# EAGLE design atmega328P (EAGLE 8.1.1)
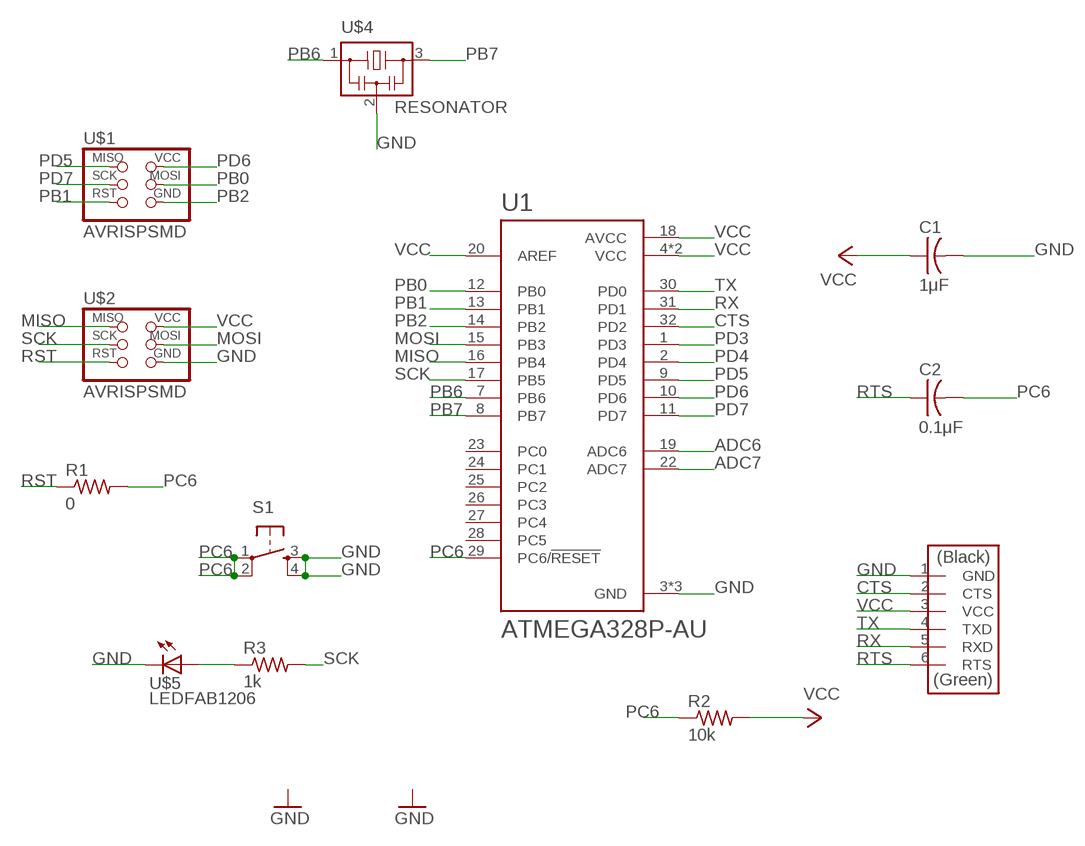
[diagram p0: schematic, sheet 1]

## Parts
C1  1μF  CAP-US1206FAB  [C1206FAB]
C2  0.1μF  CAP-US1206FAB  [C1206FAB]
R1  0  RES-US1206FAB  [R1206FAB]
R2  10k  RES-US1206FAB  [R1206FAB]
R3  1k  RES-US1206FAB  [R1206FAB]
S1  6MM_SWITCH6MM_SWITCH  [6MM_SWITCH]
U1  ATMEGA328P-AU  [QFP80P900X900X120-32N]
U$1  AVRISPSMD  [2X03SMD]
U$2  AVRISPSMD  [2X03SMD]
U$3  FTDI-SMD-HEADER  [1X06SMD]
U$4  RESONATOR  [EFOBM]
U$5  LEDFAB1206  [LED1206FAB]

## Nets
ADC6: U1.19(ADC6)
ADC7: U1.22(ADC7)
CTS: U1.32(PD2) U$3.2(CTS)
GND: C1.2 S1.3(S) S1.4(S1) U1.3(GND) U1.5(GND) U1.21(GND) U$2.6(GND) U$3.1(GND) U$4.2 U$5.2(C)
MISO: U1.16(PB4) U$2.1(MISO)
MOSI: U1.15(PB3) U$2.4(MOSI)
N$1: R3.1 U$5.1(A)
PB0: U1.12(PB0) U$1.4(MOSI)
PB1: U1.13(PB1) U$1.5(RST)
PB2: U1.14(PB2) U$1.6(GND)
PB6: U1.7(PB6) U$4.1
PB7: U1.8(PB7) U$4.3
PC6: C2.2 R1.2 R2.1 S1.1(P) S1.2(P1) U1.29(PC6/!RESET)
PD3: U1.1(PD3)
PD4: U1.2(PD4)
PD5: U1.9(PD5) U$1.1(MISO)
PD6: U1.10(PD6) U$1.2(VCC)
PD7: U1.11(PD7) U$1.3(SCK)
RST: R1.1 U$2.5(RST)
RTS: C2.1 U$3.6(RTS)
RX: U1.31(PD1) U$3.5(RXD)
SCK: R3.2 U1.17(PB5) U$2.3(SCK)
TX: U1.30(PD0) U$3.4(TXD)
VCC: C1.1 R2.2 U1.4(VCC) U1.6(VCC) U1.18(AVCC) U1.20(AREF) U$2.2(VCC) U$3.3(VCC)
Unconnected: U1.23(PC0) U1.24(PC1) U1.25(PC2) U1.26(PC3) U1.27(PC4) U1.28(PC5)

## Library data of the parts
C1 C2 = fab:CAP-US
R1-R3 = fab:RES-US: Resistor (US Symbol)
S1 = fab:6MM_SWITCH: OMRON SWITCH
U1 = ATMEGA328P-AU:ATMEGA328P-AU: ATmega Series 20 MHz 32 KB Flash 2 KB SRAM 8-Bit Microcontroller - TQFP-32; AVAILABILITY: Good; DESCRIPTION: ATmega Series 20 MHz 32 KB Flash 2 KB SRAM 8-Bit Microcontroller - TQFP-32; MF: Atmel; MP: ATMEGA328P-AU; PACKAGE: TQFP-32 Atmel; PRICE: 2.40 USD
U$1 U$2 = fab:AVRISP
U$3 = fab:FTDI-SMD-HEADER
U$4 = fab:RESONATOR
U$5 = fab:LED: LED

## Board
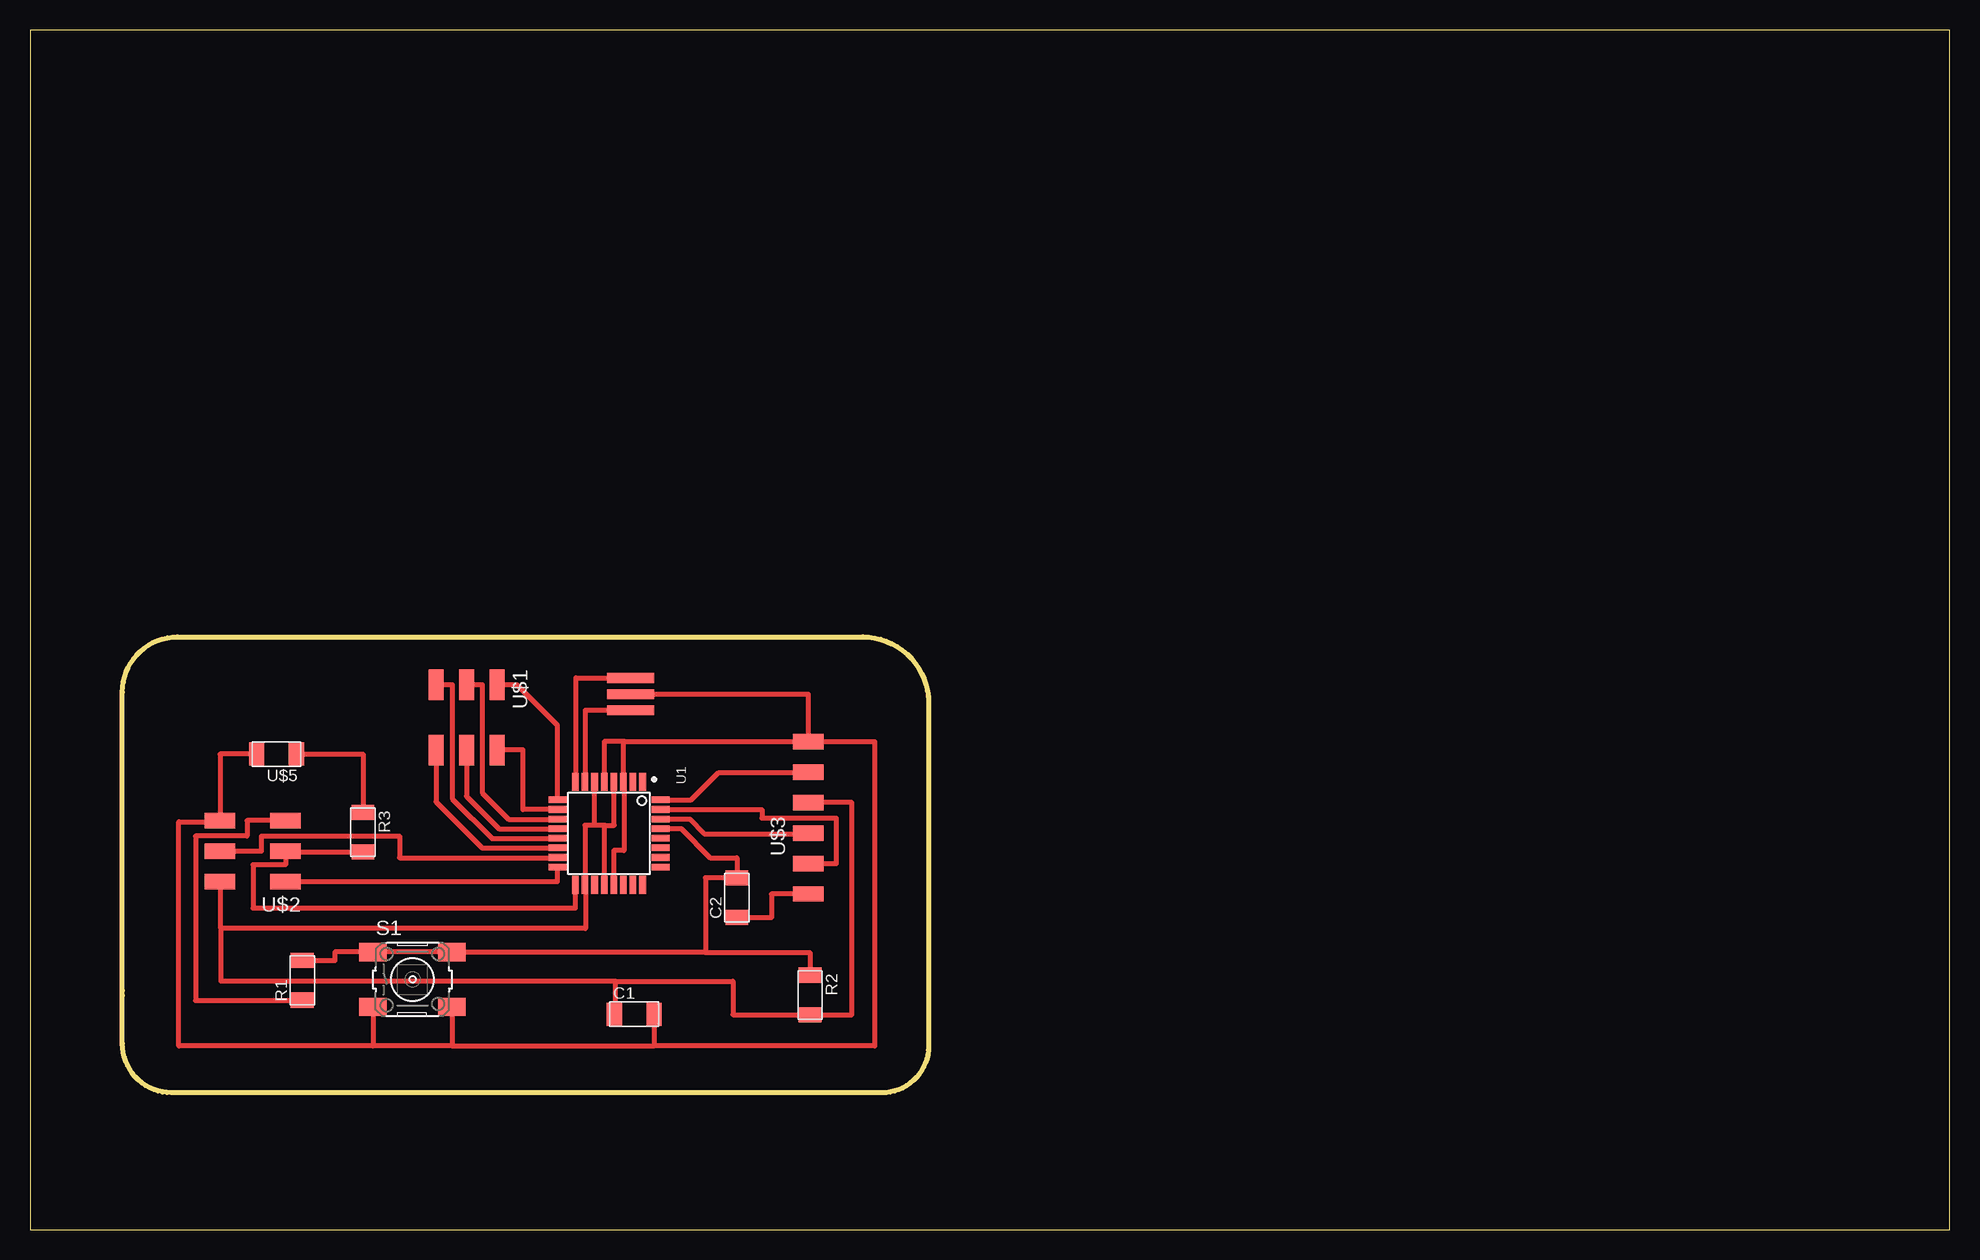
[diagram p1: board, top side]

Size 160 x 100 mm. Coordinates in mm from the lower left corner, seen from the top.
Outline: 0,0 160,0 160,100 0,100 0,0
Outline: 7.7,19.5 7.7,19.9 7.7,44.8 arc-90 12.3,49.4 69.4,49.4 arc-90 74.9,43.9 74.9,15.3 arc-90 71,11.4 11.8,11.4 arc-90 7.7,15.5 7.7,19.5
Copper layers (1*16): Top 0.035mm / dielectric 1.5mm / Bottom 0.035mm
Design rules "default": minimum track width 10mil, minimum drill 24mil, track to track 8mil, track to pad 8mil, pad to pad 8mil, via to via 8mil, smd to smd 8mil, copper to edge 40mil, drill to drill 8mil, minimum pad ring 10mil, minimum via ring 8mil, stop-mask expansion 4mil, vias tented up to drill 0mil, thermal gap 10mil

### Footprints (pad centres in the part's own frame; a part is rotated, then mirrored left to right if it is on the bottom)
C1206FAB = smd 1.27 x 1.905: 1 -1.651,0; 2 1.651,0
R1206FAB = smd 1.27 x 1.905: 1 -1.651,0; 2 1.651,0
6MM_SWITCH = smd 2.286 x 1.524: 1 -3.302,2.286; 2 3.302,2.286; 3 -3.302,-2.286; 4 3.302,-2.286
QFP80P900X900X120-32N = smd 1.5 x 0.55: 1 -4.3,2.8; 2 -4.3,2; 3 -4.3,1.2; 4 -4.3,0.4; 5 -4.3,-0.4; 6 -4.3,-1.2; 7 -4.3,-2; 8 -4.3,-2.8; 17 4.3,-2.8; 18 4.3,-2; 19 4.3,-1.2; 20 4.3,-0.4; 21 4.3,0.4; 22 4.3,1.2; 23 4.3,2; 24 4.3,2.8 | smd 0.55 x 1.5: 9 -2.8,-4.3; 10 -2,-4.3; 11 -1.2,-4.3; 12 -0.4,-4.3; 13 0.4,-4.3; 14 1.2,-4.3; 15 2,-4.3; 16 2.8,-4.3; 25 2.8,4.3; 26 2,4.3; 27 1.2,4.3; 28 0.4,4.3; 29 -0.4,4.3; 30 -1.2,4.3; 31 -2,4.3; 32 -2.8,4.3
2X03SMD = smd 2.54 x 1.27: 1 -2.54,2.54; 2 2.92,2.54; 3 -2.54,0; 4 2.92,0; 5 -2.54,-2.54; 6 2.92,-2.54
1X06SMD = smd 2.54 x 1.27: 1 0,6.35; 2 0,3.81; 3 0,1.27; 4 0,-1.27; 5 0,-3.81; 6 0,-6.35
EFOBM = smd 0.8 x 3.9: 1 -1.35,0; 2 0,0; 3 1.35,0
LED1206FAB = smd 1.27 x 1.905: 1 -1.651,0; 2 1.651,0

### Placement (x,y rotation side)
C1  50.36,17.95 0 top
C2  58.92,27.67 90 top
R1  22.7,20.78 90 top
R2  65.02,19.55 270 top
R3  27.75,33.12 270 top
S1  31.88,20.84 0 top
U1  48.26,33.02 270 top
U$1  36.39,42.89 270 top
U$2  18.77,31.55 180 top
U$3  64.87,34.32 0 top
U$4  50.06,44.63 90 top
U$5  20.55,39.64 180 top

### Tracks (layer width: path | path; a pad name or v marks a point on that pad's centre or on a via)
CTS
  Top 0.406: U$3.2 64.87,38.1 | 64.84,38.1 U$3.2 | U1.32 55.12,35.82 57.4,38.1 64.84,38.1 | 64.84,38.1 U$3.2
GND
  Top 0.406: U$5.2 15.85,39.64 U$2.6 15.85,34 12.4,34 12.4,15.3 28.6,15.3 | 52,15.3 70.4,15.3 70.4,40.67 U$3.1 | 35.2,15.3 28.6,15.3 | 35.2,15.3 52,15.3 | C1.2 52,15.3 | U1.21 48.66,31.6 49.5,31.6 49.5,37.32 U1.3 49.46,40.53 49.6,40.67 | 49.6,40.67 U$3.1 | 49.6,40.67 47.86,40.67 U1.5 | U$4.2 64.87,44.63 U$3.1 | 28.5,18.48 S1.3 28.6,18.55 28.6,15.3 | S1.4 35.2,18.55 35.2,15.3
MISO
  Top 0.406: U$2.1 43.96,29.01 U1.16
MOSI
  Top 0.406: U$2.4 19.3,31.55 19.3,32.8 30.8,32.8 30.8,31 43.96,31 U1.15
N$1
  Top 0.406: U$5.1 27.75,39.64 R3.1
PB0
  Top 0.406: U$1.4 36.39,36.11 39.1,33.4 43.94,33.4 U1.12
PB1
  Top 0.406: U$1.5 35.2,45.43 35.2,35.9 38.5,32.6 43.94,32.6 U1.13
PB2
  Top 0.406: U$1.6 33.85,35.65 37.7,31.8 43.94,31.8 U1.14
PB6
  Top 0.406: 46.3,37.32 U1.7 46.3,37.32 | 46.3,37.32 46.3,43.3 50.06,43.3 U$4.1
PB7
  Top 0.406: 45.4,37.32 U1.8 45.5,37.32 45.5,46 50.06,46 U$4.3
PC6
  Top 0.406: U1.29 54.28,33.42 56.7,31 58.92,31 C2.2 56.3,29.32 56.3,23.1 | 56.3,23.1 65.02,23.1 R2.1 | 56.3,23.1 35.18,23.1 S1.2 S1.1 25.4,23.13 25.4,22.4 22.7,22.4 R1.2
PD5
  Top 0.406: 44,35.86 U1.9 43.96,42.04 40.6,45.4 38.96,45.4 U$1.1
PD6
  Top 0.406: U1.10 41.1,35.02 41.1,40 38.93,40 U$1.2
PD7
  Top 0.406: U$1.3 37.7,45.43 37.7,36.4 39.9,34.2 43.94,34.2 U1.11
RST
  Top 0.406: U$2.5 18.1,34.09 18.1,32.8 13.8,32.8 13.8,19.1 22.7,19.1 R1.1
RTS
  Top 0.406: U$3.6 61.8,27.97 61.8,26 58.92,26 C2.1
RX
  Top 0.406: U1.31 61,35.02 61,34.3 67.2,34.3 67.2,30.5 U$3.5
SCK
  Top 0.406: R3.2 21.39,31.47 U$2.3 21.3,30.4 18.6,30.4 18.6,26.8 45.46,26.8 U1.17
TX
  Top 0.406: 52.56,34.2 U1.30 54.98,34.22 56.2,33 64.82,33 U$3.4
VCC
  Top 0.406: U$3.3 68.5,35.59 68.5,17.9 R2.2 58.6,17.9 58.6,20.7 48.8,20.7 | U$2.2 15.9,29.01 15.9,25.1 | 48.8,20.7 15.9,20.7 15.9,25.1 | C1.1 48.8,17.95 48.8,20.7 | 15.9,25.1 46.3,25.1 46.3,28.72 U1.18 46.26,33.7 47,33.7 | 47.1,37.32 U1.6 47,37.32 47,33.7 | 48.7,37.32 U1.4 48.66,33.74 48.7,33.7 47.9,33.7 | 47.9,33.7 47,33.7 | U1.20 47.9,28.72 47.9,33.7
